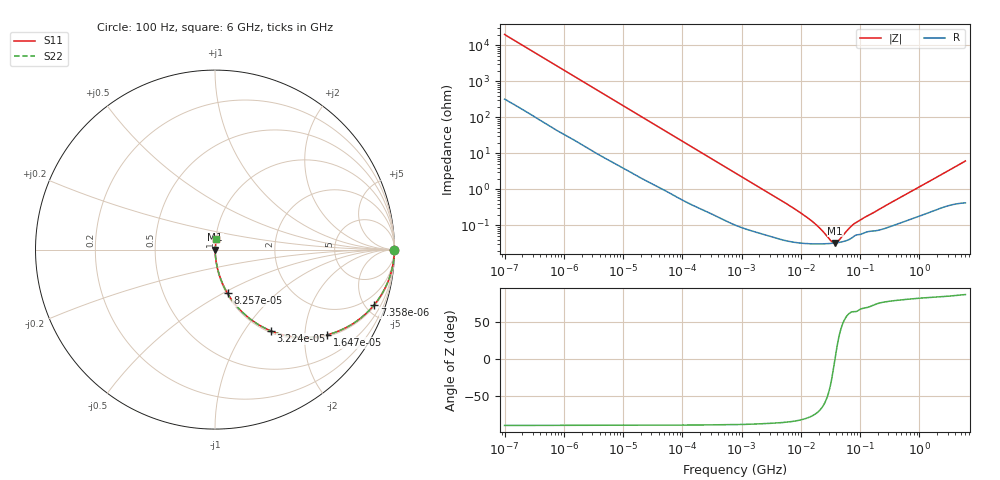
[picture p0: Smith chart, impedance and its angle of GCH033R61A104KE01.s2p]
!Murata Part Number: GCH033R61A104KE01
!These Parameters are Measured in Series Mode Connection
!Data Generated on Jun 19, 2026
!  o--ll--o
!Port1  Port2
!  o------o
!Operation Temp=25[degC], DC Bias Voltage=0[V]
!Freq. Start=100[Hz] Stop=6[GHz] 401[Steps]
# Hz S RI R 50
!Freq.(Hz) S11(Real) S11(Imag) S21(Real) S21(Imag) S12(Real) S12(Imag) S22(Real) S22(Imag)
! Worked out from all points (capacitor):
!   401 points, 100 Hz to 6 GHz, reference 50 ohm
!   read as one part in series: C = 78.5 nF near 109 Hz
!   lowest |Z| = 32.5 mohm at 38.09 MHz (marker M1)
!   series resonance near 37.8 MHz, so ESL is about 230 pH
!   S11 on the Smith chart (normalised r, x): 100 Hz: open; 7.358 kHz: 1.10, -5.74; 16.47 kHz: 1.05, -2.59; 32.24 kHz: 1.03, -1.33; 82.57 kHz: 1.01, -0.53; 6 GHz: 1.01, +0.12
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100  0.9999 -0.00495  0.000104 0.00495  0.000104 0.00495  0.9999 -0.00495
627  0.9986 -0.0304  0.00141 0.0304  0.00141 0.0304  0.9986 -0.0304
2008  0.9892 -0.0952  0.0108 0.0952  0.0108 0.0952  0.9892 -0.0952
4299  0.9567 -0.1951  0.0433 0.1951  0.0433 0.1951  0.9567 -0.1951
7358  0.8875 -0.3071  0.1125 0.3071  0.1125 0.3071  0.8875 -0.3071
11009  0.7837 -0.4025  0.2163 0.4025  0.2163 0.4025  0.7837 -0.4025
16473  0.6241 -0.4749  0.3759 0.4749  0.3759 0.4749  0.6241 -0.4749
22537  0.4748 -0.4896  0.5252 0.4896  0.5252 0.4896  0.4748 -0.4896
32244  0.3113 -0.4528  0.6887 0.4528  0.6887 0.4528  0.3113 -0.4528
40335  0.2271 -0.4084  0.7729 0.4084  0.7729 0.4084  0.2271 -0.4084
82567  0.0699 -0.2438  0.9301 0.2438  0.9301 0.2438  0.0699 -0.2438
221108  0.0125 -0.0983  0.9875 0.0983  0.9875 0.0983  0.0125 -0.0983
774597  0.00187 -0.029  0.9981 0.029  0.9981 0.029  0.00187 -0.029
6353432  0.000372 -0.00359  0.9996 0.00359  0.9996 0.00359  0.000372 -0.00359
1.555665e7  0.000309 -0.00126  0.9997 0.00126  0.9997 0.00126  0.000309 -0.00126
2.225763e7  0.000307 -0.000693  0.9997 0.000693  0.9997 0.000693  0.000307 -0.000693
3.184506e7  0.000316 -0.000215  0.9997 0.000215  0.9997 0.000215  0.000316 -0.000215
3.80911e7  0.000325 9.7e-06  0.9997 -9.7e-06  0.9997 -9.7e-06  0.000325 9.7e-06
4.35672e7  0.000336 0.000178  0.9997 -0.000178  0.9997 -0.000178  0.000336 0.000178
7.797396e7  0.000492 0.00097  0.9995 -0.00097  0.9995 -0.00097  0.000492 0.00097
3.124326e8  0.000923 0.00396  0.9991 -0.00396  0.9991 -0.00396  0.000923 0.00396
6e9  0.00796 0.0609  0.992 -0.0609  0.992 -0.0609  0.00796 0.0609
